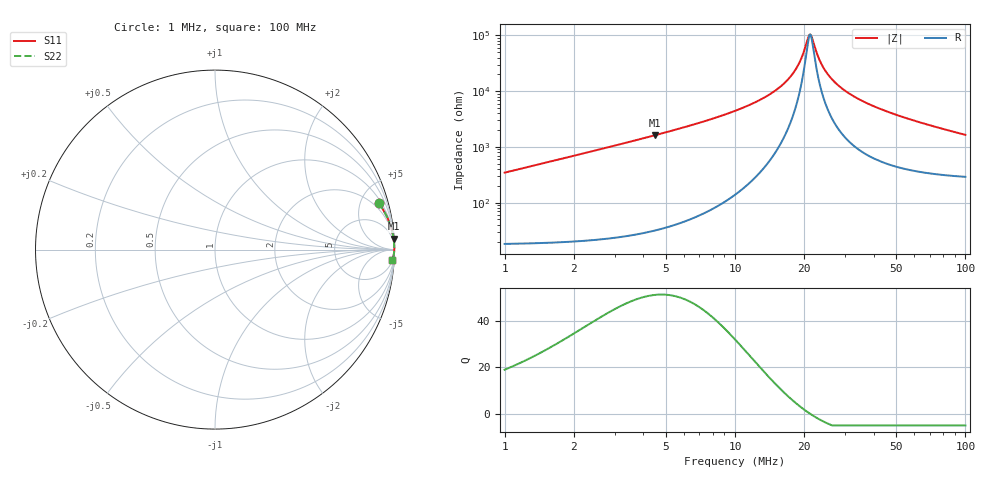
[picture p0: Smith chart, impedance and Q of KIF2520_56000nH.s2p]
!version-2
!date-12.2020
!Series
# MHz S RI R 50
!Freq ReS11 ImS11 ReS21 ImS21 ReS12 ImS12 ReS22 ImS22
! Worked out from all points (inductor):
!   991 points, 1 MHz to 100 MHz, reference 50 ohm
!   read as one part in series: L = 54.8 uH near 1.4 MHz
!   highest Q = 50.9 at 4.5 MHz (marker M1), where L = 57.4 uH
!   self-resonance near 21.1 MHz
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1  0.9111 0.2595  0.0889 -0.2595  0.0889 -0.2595  0.9111 0.2595
2.5  0.9843 0.1124  0.0157 -0.1124  0.0157 -0.1124  0.9843 0.1124
4.5  0.995 0.0613  0.00497 -0.0613  0.00497 -0.0613  0.995 0.0613
7.2  0.9979 0.0356  0.00206 -0.0356  0.00206 -0.0356  0.9979 0.0356
14.4  0.9991 0.0108  0.000861 -0.0108  0.000861 -0.0108  0.9991 0.0108
17.5  0.9991 0.00527  0.000853 -0.00527  0.000853 -0.00527  0.9991 0.00527
19  0.9991 0.003  0.000885 -0.003  0.000885 -0.003  0.9991 0.003
19.7  0.9991 0.002  0.000906 -0.002  0.000906 -0.002  0.9991 0.002
20.7  0.9991 0.00065  0.000942 -0.00065  0.000942 -0.00065  0.9991 0.00065
21.2  0.999 -1.83e-06  0.000962 1.83e-06  0.000962 1.83e-06  0.999 -1.83e-06
21.6  0.999 -0.000512  0.000979 0.000512  0.000979 0.000512  0.999 -0.000512
22.7  0.999 -0.00187  0.00103 0.00187  0.00103 0.00187  0.999 -0.00187
23.5  0.9989 -0.00282  0.00107 0.00282  0.00107 0.00282  0.9989 -0.00282
24.5  0.9989 -0.00396  0.00113 0.00396  0.00113 0.00396  0.9989 -0.00396
25.6  0.9988 -0.00518  0.0012 0.00518  0.0012 0.00518  0.9988 -0.00518
29.1  0.9986 -0.00878  0.00144 0.00878  0.00144 0.00878  0.9986 -0.00878
34  0.9981 -0.0133  0.00187 0.0133  0.00187 0.0133  0.9981 -0.0133
41  0.9974 -0.0192  0.00262 0.0192  0.00262 0.0192  0.9974 -0.0192
50.5  0.9962 -0.0265  0.00385 0.0265  0.00385 0.0265  0.9962 -0.0265
67  0.9934 -0.038  0.00659 0.038  0.00659 0.038  0.9934 -0.038
83.5  0.99 -0.0485  0.01 0.0485  0.01 0.0485  0.99 -0.0485
100  0.986 -0.0583  0.014 0.0583  0.014 0.0583  0.986 -0.0583
